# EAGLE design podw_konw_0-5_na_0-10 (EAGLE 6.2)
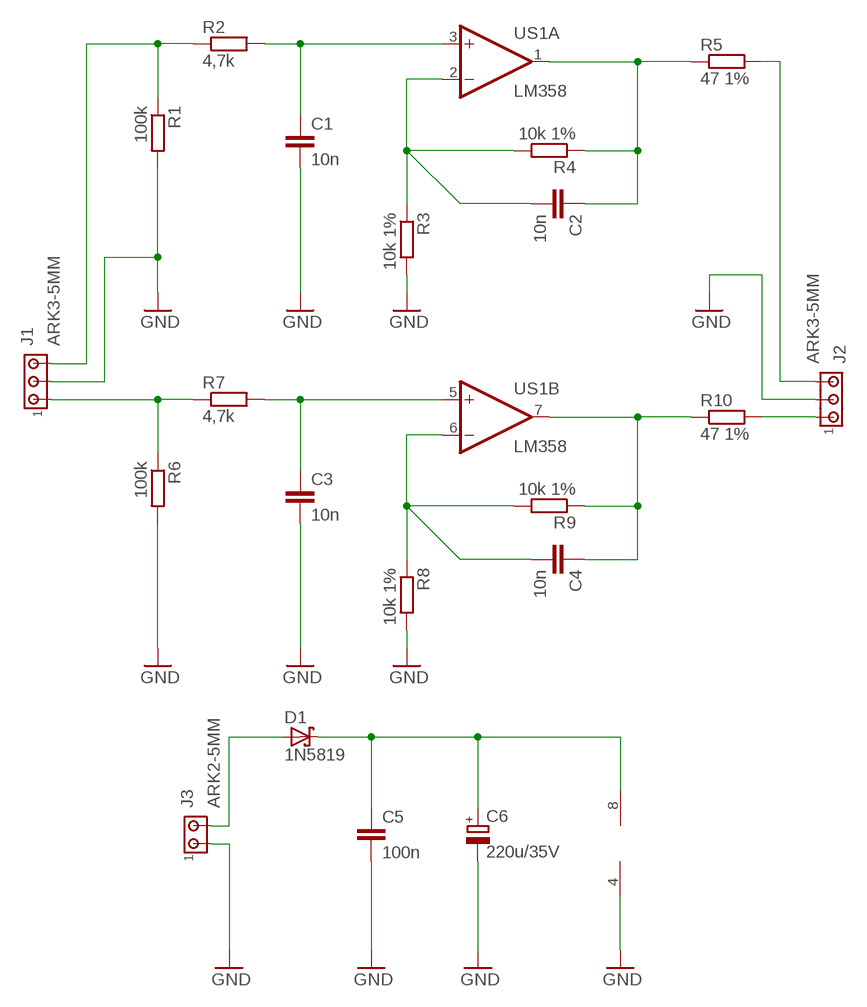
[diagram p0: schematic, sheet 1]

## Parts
C1  10n  C-EU050-025X075  [C050-025X075]
C2  10n  C-EU050-025X075  [C050-025X075]
C3  10n  C-EU050-025X075  [C050-025X075]
C4  10n  C-EU050-025X075  [C050-025X075]
C5  100n  C-EU050-025X075  [C050-025X075]
C6  220u/35V  CPOL-EUE3.5-8  [E3,5-8]
D1  1N5819  1N5819-T  [DO41-7.6]
J1  ARK3-5MM  [3PIN-5MM]
J2  ARK3-5MM  [3PIN-5MM]
J3  ARK2-5MM  [2PIN-5MM]
R1  100k  R-EU_0207/7  [0207/7]
R2  4,7k  R-EU_0207/7  [0207/7]
R3  10k 1%  R-EU_0207/7  [0207/7]
R4  10k 1%  R-EU_0207/7  [0207/7]
R5  47 1%  R-EU_0207/7  [0207/7]
R6  100k  R-EU_0207/7  [0207/7]
R7  4,7k  R-EU_0207/7  [0207/7]
R8  10k 1%  R-EU_0207/7  [0207/7]
R9  10k 1%  R-EU_0207/7  [0207/7]
R10  47 1%  R-EU_0207/7  [0207/7]
US1  LM358  LM358N  [DIL08]

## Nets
GND: C1.2 C3.2 C5.2 C6.- J1.P$2 J2.P$2 J3.P$1 R1.2 R3.2 R6.2 R8.2 US1.4(P:V-)
N$1: J1.P$3 R1.1 R2.1
N$2: C1.1 R2.2 US1.3(A:+IN)
N$3: C2.1 R4.1 R5.1 US1.1(A:OUT)
N$4: C2.2 R3.1 R4.2 US1.2(A:-IN)
N$5: J2.P$3 R5.2
N$6: C5.1 C6.+ D1.C US1.8(P:V+)
N$7: C3.1 R7.2 US1.5(B:+IN)
N$8: C4.1 R9.1 R10.1 US1.7(B:OUT)
N$9: C4.2 R8.1 R9.2 US1.6(B:-IN)
N$10: J1.P$1 R6.1 R7.1
N$11: J2.P$1 R10.2
N$18: D1.A J3.P$2

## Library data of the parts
C1-C5 = rcl:C-EU: CAPACITOR, European symbol
C6 = rcl:CPOL-EU: POLARIZED CAPACITOR, European symbol
D1 = diode:1N581*: 1.0A SCHOTTKY BARRIER RECTIFIER
J1 J2 = zlacza_futrzak:ARK3: ARK 3 Raster 5mm i 3,5mm
J3 = zlacza_futrzak:ARK2: ARK 2
R1-R10 = rcl:R-EU_: RESISTOR, European symbol
US1 = linear:LM358: OP AMP also LM158; LM258; LM2904 Source: http://cache.national.com/ds/LM/LM158.pdf

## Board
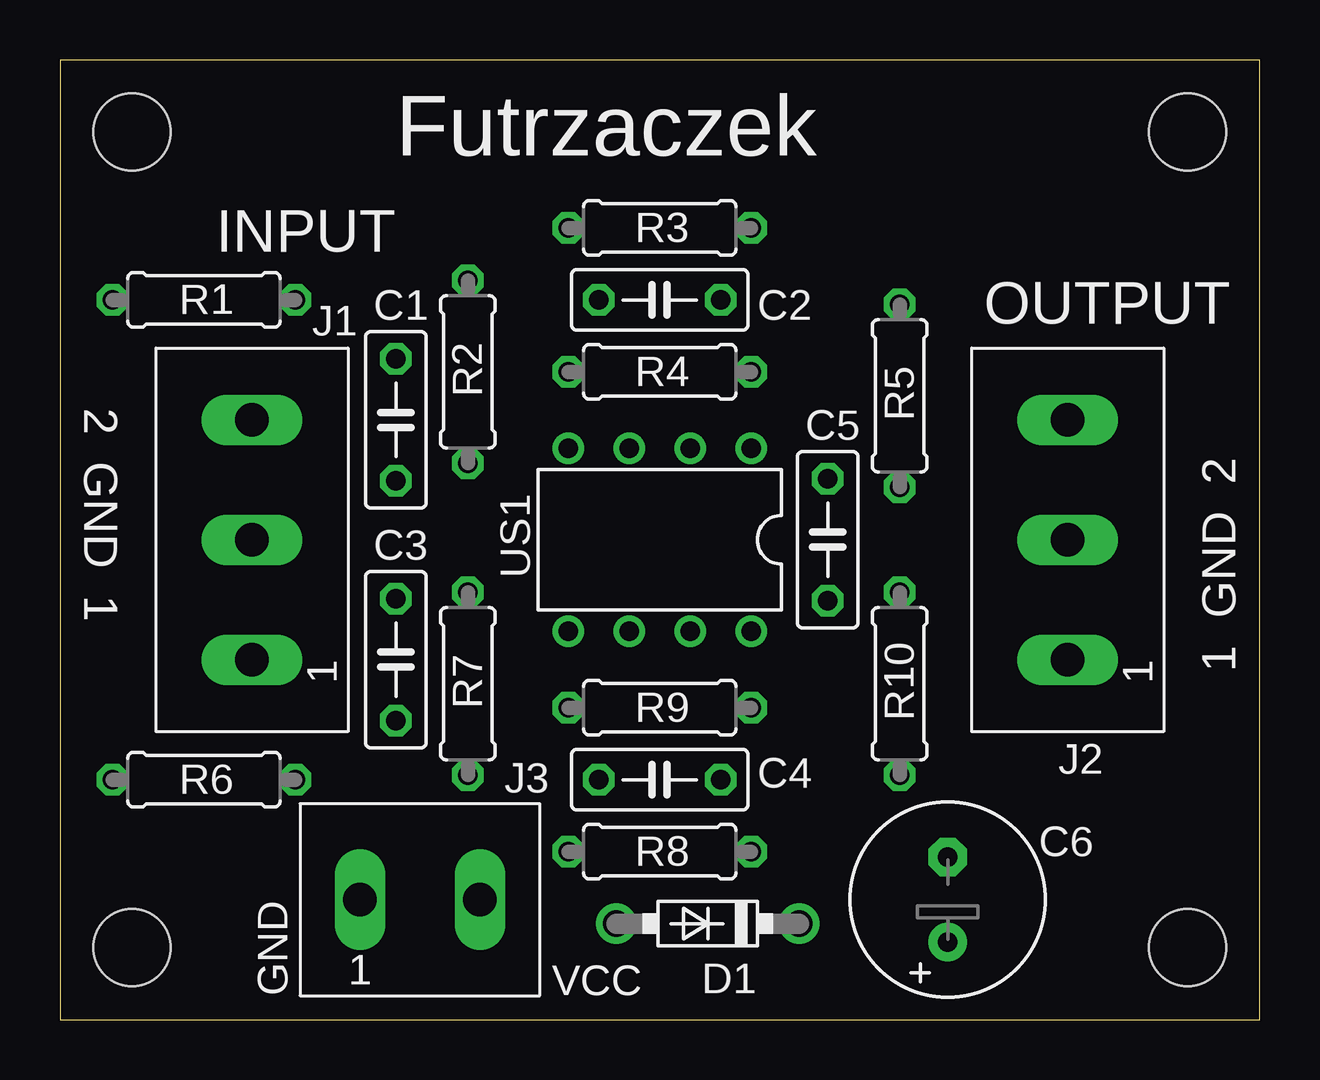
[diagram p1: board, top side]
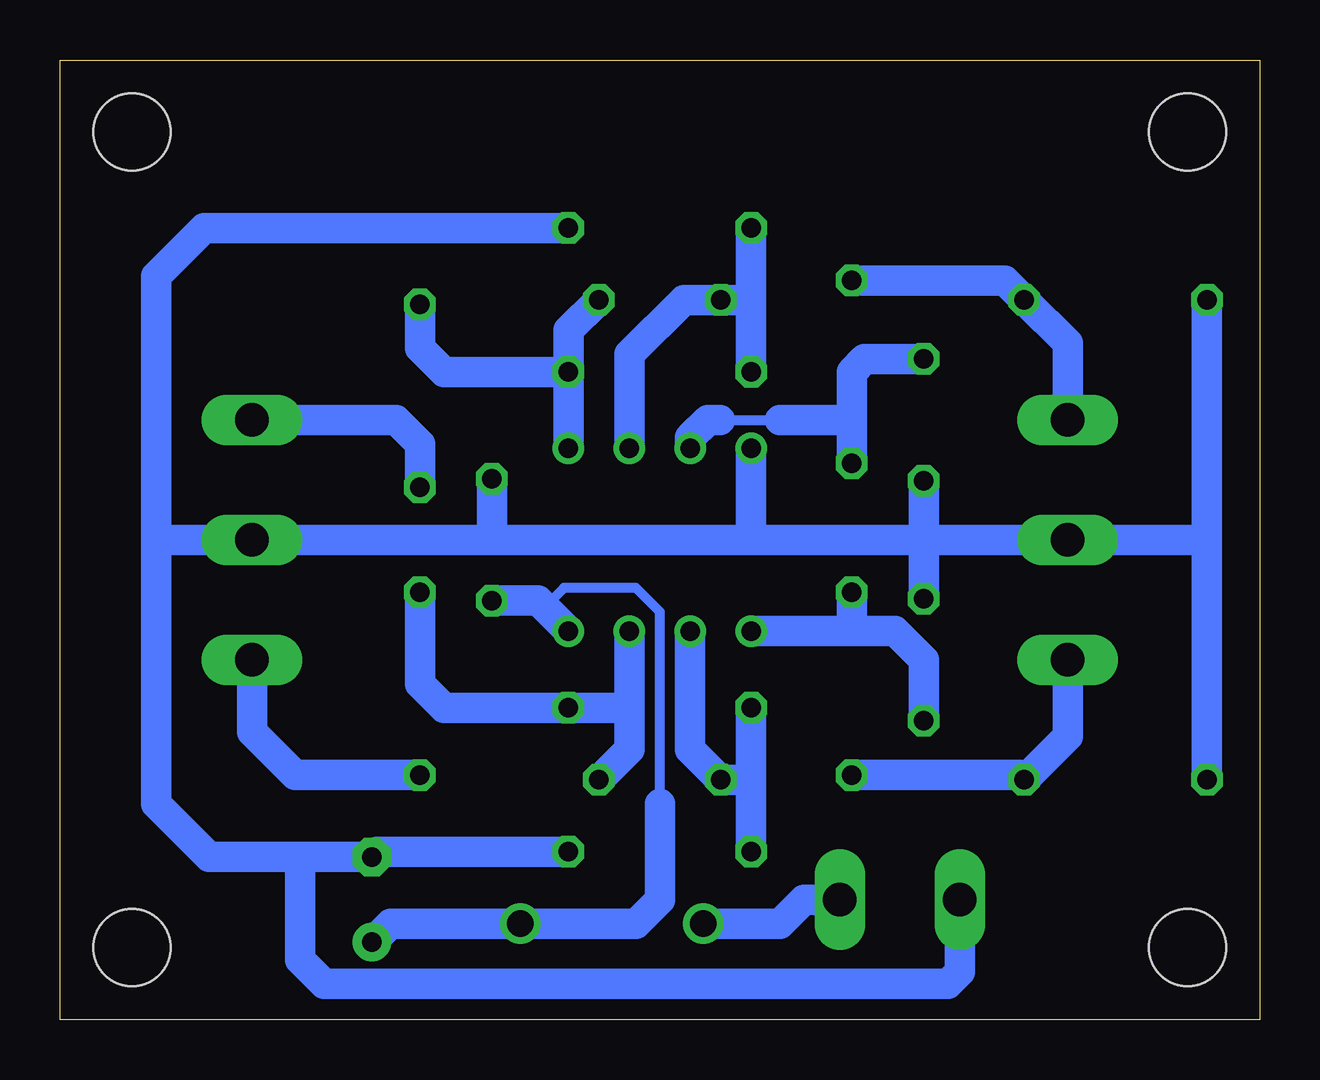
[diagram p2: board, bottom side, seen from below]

Size 50 x 40 mm. Coordinates in mm from the lower left corner, seen from the top.
Outline: 0,0 50,0 50,40 0,40 0,0
Copper layers (1*16): Top 0.035mm / dielectric 1.5mm / Bottom 0.035mm
Design rules: minimum track width 10mil, minimum drill 24mil, track to track 8mil, track to pad 8mil, pad to pad 8mil, via to via 8mil, smd to smd 8mil, copper to edge 20mil, drill to drill 8mil, minimum pad ring 10mil, minimum via ring 8mil, stop-mask expansion 4mil, vias tented up to drill 0mil, thermal gap 10mil
Holes 3.2 mm at 3,3 3,37 47,3 47,37

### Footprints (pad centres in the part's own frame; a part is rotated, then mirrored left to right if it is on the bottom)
C050-025X075 = drill 0.813 octagon: 1 -2.54,0; 2 2.54,0
E3,5-8 = drill 0.813 pad 1.6: + -1.778,0 | drill 0.813 pad 1.6 octagon: - 1.778,0
DO41-7.6 = drill 1.1 pad 1.7: A 3.81,0; C -3.81,0
3PIN-5MM = drill 1.4 long: P$1 -5,0; P$2 0,0; P$3 5,0
2PIN-5MM = drill 1.4 long: P$1 -2.5,0; P$2 2.5,0
0207/7 = drill 0.813 octagon: 1 -3.81,0; 2 3.81,0
DIL08 = drill 0.813 pad 1.27: 1 -3.81,-3.81; 2 -1.27,-3.81; 3 1.27,-3.81; 4 3.81,-3.81; 5 3.81,3.81; 6 1.27,3.81; 7 -1.27,3.81; 8 -3.81,3.81

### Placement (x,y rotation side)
C1  14,25 270 top
C2  25,30 180 top
C3  14,15 90 top
C4  25,10 180 top
C5  32,20 90 top
C6  37,5 90 top
D1  27,4 180 top
J1  8,20 90 top
J2  42,20 90 top
J3  15,5 0 top
R1  6,30 180 top
R2  17,27 270 top
R3  25,33 0 top
R4  25,27 180 top
R5  35,26 270 top
R6  6,10 180 top
R7  17,14 90 top
R8  25,7 0 top
R9  25,13 180 top
R10  35,14 270 top
US1  25,20 180 top

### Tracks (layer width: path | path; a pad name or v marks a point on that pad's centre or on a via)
GND
  Bottom 1.27: R6.2 2.19,20 | 2.19,20 R1.2 | 2.19,20 J1.P$2 14,20 | 14,20 21,20 | 21,20 32,20 | 32,20 J2.P$2 45,20 46,20 | C3.2 14,20 | C1.2 14,20 | US1.4 21.19,20.19 21,20 | R3.2 44,33 46,31 46,21 46,20 | C5.2 32,20 | 40,6.78 C6.- 36.78,7 R8.2 | 40,6.78 43.78,6.78 45,8 46,9 46,20 | J3.P$1 12.5,2 13,1.5 34.5,1.5 35,1.5 39,1.5 40,2.5 40,6.78
N$1
  Bottom 1.27: J1.P$3 8,28.19 R1.1 10.62,30.81 R2.1
N$2
  Bottom 0.406: 22.5,25 20,25
  Bottom 1.27: C1.1 16.46,27.54 17,27 17,25 | 17,25 R2.2 | US1.3 23.73,24.27 23,25 22.5,25 | 17,25 20,25
N$3
  Bottom 1.27: US1.1 R4.1 | R4.1 28.81,28.73 C2.1 | R4.1 34,27 35,28 R5.1
N$4
  Bottom 1.27: US1.2 26.27,27.73 24,30 C2.2 21.19,30 | R4.2 21.19,30 | 21.19,30 R3.1
N$5
  Bottom 1.27: R5.2 35,24 36,25 J2.P$3
N$6
  Bottom 0.406: 25,9 25,17 26,18 29,18 29.81,17.19
  Bottom 1.27: C5.1 30.08,17.46 29.81,17.19 US1.8 | 25,9 25,5 26,4 D1.C 36.22,4 C6.+
N$7
  Bottom 1.27: US1.5 17,16.19 | 17,16.19 15.19,16.19 14,15 C3.1 | R7.2 17,16.19
N$8
  Bottom 1.27: R10.1 35,14 34,13 R9.1 26.27,13 | US1.7 26.27,13 | 26.27,13 26.27,11.27 C4.1
N$9
  Bottom 1.27: US1.6 23.73,11.27 C4.2 21.19,10 R9.2 R8.1
N$10
  Bottom 1.27: R7.1 10,10.19 R6.1 8,11.81 J1.P$1
N$11
  Bottom 1.27: R10.2 40.19,10.19 42,12 J2.P$1
N$18
  Bottom 1.27: D1.A 20,4 19,5 J3.P$2

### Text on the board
tPlace: Futrzaczek | INPUT | OUTPUT | 2 GND 1 | 1 GND 2 | GND | VCC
